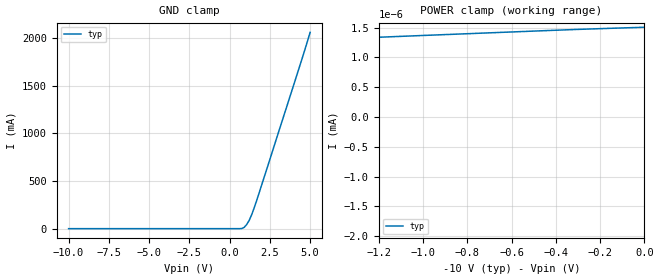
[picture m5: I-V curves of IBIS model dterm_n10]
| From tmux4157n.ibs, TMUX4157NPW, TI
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| dterm_n10
[Model]   dterm_n10
Model_type   Terminator
|   typ   min   max
C_comp   1.457606e-11   NA   NA
[Voltage Range]   -10   NA   NA
[Temperature Range]   27   NA   NA
[Power Clamp Reference]   -10   NA   NA
[GND Clamp Reference]   0   NA   NA
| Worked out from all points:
|   POWER clamp passes 1 mA (typ) near -10.71 V on its own axis
[GND Clamp]
|   Voltage   I(typ)   I(min)   I(max)
-10V      -1.028nA   NA         NA
606.1mV   145.4uA    NA         NA
909.1mV   13.77mA    NA         NA
1.212V    84.88mA    NA         NA
1.364V    143.7mA    NA         NA
1.667V    288.1mA    NA         NA
4.394V    1.728A     NA         NA
5V        2.06A      NA         NA
[POWER Clamp]
|   Voltage   I(typ)   I(min)   I(max)
-15V      -2.157A    NA         NA
-10.3V    -28.91nA   NA         NA
-10.15V   -1.237nA   NA         NA
-10V      -1.028nA   NA         NA
-8.182V   -584.7pA   NA         NA
-5.455V   4.909pA    NA         NA
-5.152V   139pA      NA         NA
-5V       246.4pA    NA         NA
-4.545V   756.9pA    NA         NA
-4.394V   816.5pA    NA         NA
-2.424V   1.152nA    NA         NA
0V        1.506nA    NA         NA
